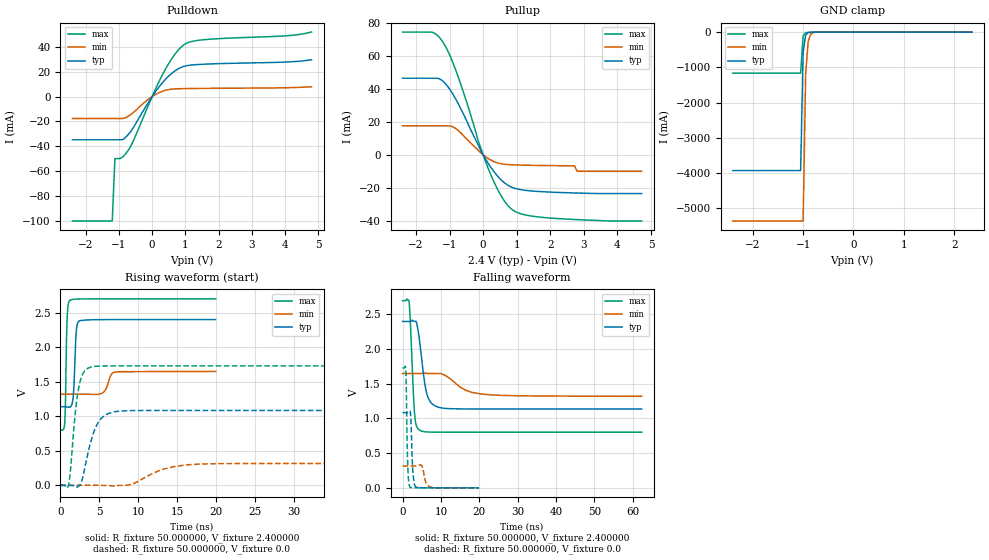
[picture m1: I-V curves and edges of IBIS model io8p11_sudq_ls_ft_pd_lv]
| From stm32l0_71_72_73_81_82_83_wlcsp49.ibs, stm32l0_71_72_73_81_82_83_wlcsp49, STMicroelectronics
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|   Model io8p11_sudq_ls_ft_pd_lv
[Model]  io8p11_sudq_ls_ft_pd_lv
Model_type I/O
Polarity   Non-Inverting
Enable   Active-Low
Vinl =   0.720000V
Vinh =   1.680000V
Vmeas =  1.200000V
Cref =   50.000000pF
Rref =   100.000000M
Vref =   0.0V
C_comp   2.317700pF   2.286600pF   2.332700pF
[Temperature Range]   25.000000   0.105000k   -40.000000
[Pullup Reference]   2.400000V   1.650000V   2.700000V
[Pulldown Reference]   0.0V   0.0V   0.0V
[POWER Clamp Reference]   2.400000V   1.650000V   2.700000V
[GND Clamp Reference]   0.0V   0.0V   0.0V
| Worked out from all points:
|   slope of the pulldown table from 0 to 0.36 V, typ, clamps not added: 28.4 ohm
|   slope of the pullup table from 0 to 0.36 V, typ, clamps not added: 32.2 ohm
|   GND clamp passes 1 mA (typ) near -0.64 V on its own axis
|   rising waveform, R_fixture 50.000000, V_fixture 2.400000: 20-80 % time 278ps typ, 638ps min, 187ps max; typ from 1.14 V to 2.4 V
|   rising waveform, R_fixture 50.000000, V_fixture 0.0: 20-80 % time 1.58ns typ, 3.85ns min, 919ps max; typ from 0 V to 1.08 V
|   falling waveform, R_fixture 50.000000, V_fixture 2.400000: 20-80 % time 1.81ns typ, 5.39ns min, 912ps max; typ from 2.4 V to 1.14 V
|   falling waveform, R_fixture 50.000000, V_fixture 0.0: 20-80 % time 460ps typ, 843ps min, 358ps max; typ from 1.08 V to 0 V
[Pulldown]
|Voltage   I(typ)   I(min)   I(max)
-2.4V     -34.71mA   -17.62mA   -100mA
-1.2V     -34.71mA   -17.62mA   -100mA
-1.12V    -34.71mA   -17.62mA   -49.77mA
-960mV    -34.71mA   -17.62mA   -49.77mA
-720mV    -30.52mA   -15.81mA   -43.23mA
-560mV    -24.66mA   -12.69mA   -35.3mA
-80mV     -3.3mA     -1.497mA   -4.982mA
320mV     11.47mA    4.39mA     18.08mA
640mV     19.72mA    6.139mA    32.34mA
960mV     24.33mA    6.432mA    41.77mA
1.52V     26.01mA    6.613mA    45.64mA
4.8V      29.64mA    7.944mA    51.92mA
[Pullup]
|Voltage   I(typ)   I(min)   I(max)
-2.4V     46.57mA    17.61mA    74.62mA
-1.52V    46.57mA    17.61mA    74.5mA
-1.2V     44.84mA    17.61mA    68.61mA
-800mV    33.3mA     15.72mA    50.64mA
-160mV    6.59mA     3.051mA    9.467mA
240mV     -7.917mA   -3.299mA   -12.65mA
560mV     -15.67mA   -5.496mA   -25.76mA
880mV     -19.92mA   -6.062mA   -33.51mA
1.92V     -22.56mA   -6.511mA   -38.27mA
2.72V     -23.16mA   -6.64mA    -39.27mA
2.8V      -23.2mA    -10mA      -39.35mA
4.72V     -23.5mA    -10mA      -40.2mA
[GND_clamp]
|Voltage   I(typ)   I(min)   I(max)
-2.4V     -3.929A    -5.359A    -1.166A
-1.05V    -3.929A    -5.359A    -1.166A
-1V       -574.5mA   -5.359A    -109.1mA
-950mV    -90.03mA   -1.192A    -18.56mA
-900mV    -18.42mA   -269.7mA   -9.058mA
-850mV    -6.777mA   -63.61mA   -6.588mA
-800mV    -4.039mA   -16.67mA   -4.867mA
-650mV    -1.055mA   -1.235mA   -1.154mA
2.35V     52.69uA    50.02uA    36.84uA
[POWER_clamp]
|Voltage   I(typ)   I(min)   I(max)
-2.4V     0A         0A         0A
0V        0A         0A         0A
[Ramp]
| variable   typ   min   max
dV/dt_r  0.65004/1.57621n   0.18967/3.84232n   1.03746/0.91392n
dV/dt_f  0.75708/1.80566n   0.19626/5.37533n   1.13771/0.91075n
R_load = 50.000000
[Rising Waveform]
R_fixture= 50.000000
V_fixture= 2.400000
V_fixture_min= 1.650000
V_fixture_max= 2.700000
|time   V(typ)   V(min)   V(max)
0s        1.137V     1.32V      802.2mV
560.6ps   1.137V     1.32V      920.1mV
840.8ps   1.133V     1.32V      2.377V
1.201ns   1.132V     1.32V      2.678V
1.642ns   1.288V     1.32V      2.692V
2.042ns   2.241V     1.32V      2.696V
2.402ns   2.379V     1.32V      2.698V
5.365ns   2.398V     1.335V     2.699V
7.087ns   2.399V     1.639V     2.699V
19.94ns   2.399V     1.649V     2.699V
[Rising Waveform]
R_fixture= 50.000000
V_fixture= 0.0
V_fixture_min= 0.0
V_fixture_max= 0.0
|time   V(typ)   V(min)   V(max)
0s        -3.078uV   4.619uV    228.2uV
1.001ns   110.3uV    1.163uV    -14.54mV
1.251ns   -727uV     -1.743uV   171.6mV
2.002ns   -17.33mV   -4.742uV   1.146V
2.377ns   -8.004mV   11.89uV    1.429V
4.004ns   674.7mV    90.72uV    1.714V
5.38ns    984mV      -1.53mV    1.727V
7.508ns   1.073V     -1.957mV   1.729V
17.89ns   1.083V     307.2mV    1.729V
62.31ns   1.083V     316.1mV    1.729V
[Falling Waveform]
R_fixture= 50.000000
V_fixture= 2.400000
V_fixture_min= 1.650000
V_fixture_max= 2.700000
|time   V(typ)   V(min)   V(max)
0s        2.399V     1.649V     2.699V
1.752ns   2.398V     1.649V     2.658V
3.128ns   2.402V     1.649V     1.078V
3.629ns   2.385V     1.649V     893.6mV
4.505ns   2.087V     1.648V     830mV
5.756ns   1.516V     1.656V     809.4mV
6.381ns   1.345V     1.65V      806.1mV
9.384ns   1.162V     1.648V     802.5mV
20.77ns   1.138V     1.352V     802.2mV
62.31ns   1.137V     1.32V      802.2mV
[Falling Waveform]
R_fixture= 50.000000
V_fixture= 0.0
V_fixture_min= 0.0
V_fixture_max= 0.0
|time   V(typ)   V(min)   V(max)
0s        1.083V     316.1mV    1.729V
840.8ps   1.083V     316.1mV    1.708V
1.361ns   1.083V     316.1mV    323.6mV
1.922ns   1.11V      316.1mV    13.84mV
2.202ns   960.8mV    316.1mV    3.539mV
2.683ns   247.9mV    315.9mV    1.956mV
3.363ns   19.25mV    315.9mV    1.251mV
4.925ns   1.474mV    325.8mV    482.6uV
7.648ns   344.9uV    5.126mV    245.1uV
19.94ns   -3.078uV   4.619uV    228.2uV
